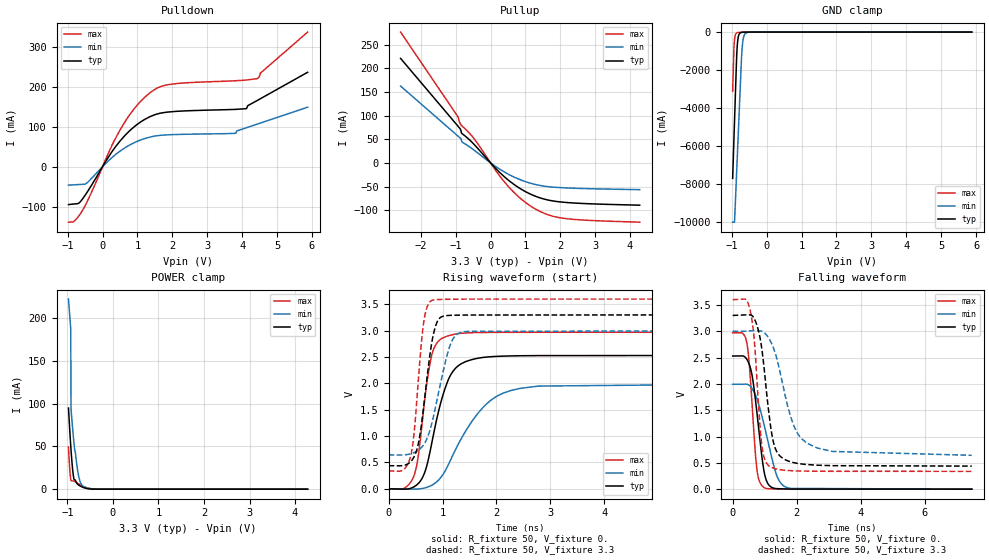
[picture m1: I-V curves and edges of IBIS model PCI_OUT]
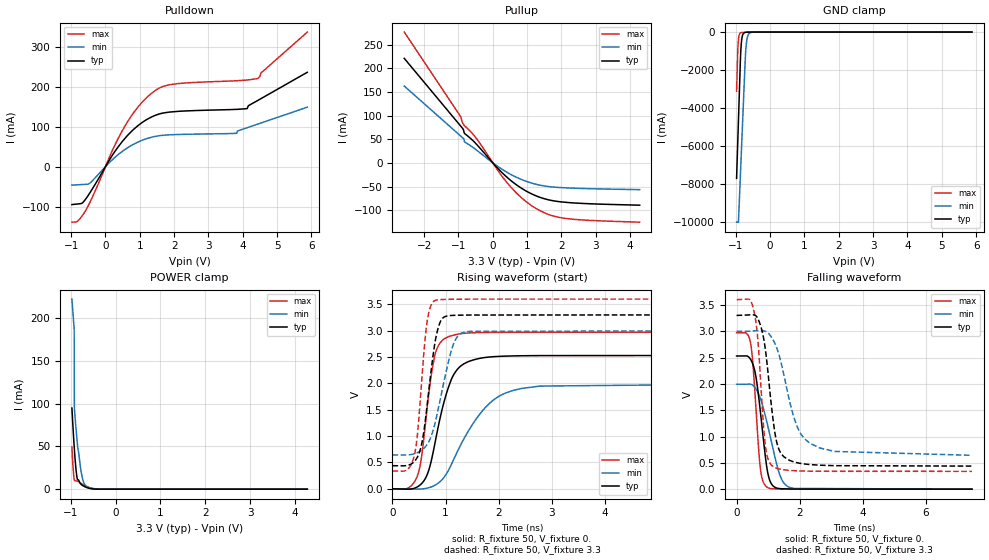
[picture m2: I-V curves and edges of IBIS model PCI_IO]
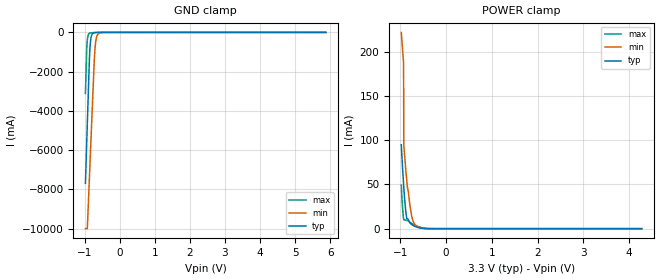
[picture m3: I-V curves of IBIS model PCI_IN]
|   IBIS Model for Tsi382 LQFP Package
[IBIS Ver]   3.2
[Disclaimer] This model is subject to change.
   Integrated Device Technology, Inc. ("IDT") hereby grants the
   user of this IBIS model a non-exclusive, nontransferable
   license to use this IBIS model under the following terms. The
   user is granted this license only to use the IBIS model and is
   not granted rights to sell, copy (except as needed to run the
   IBIS model), rent, lease or sub-license the IBIS model in
   whole or in part, or in modified form to anyone. The User may
   modify the IBIS model to suit its specific applications, but
   rights to derivative works and such modifications shall belong
   to IDT. This IBIS model is provided on an AS IS" basis and IDT
   makes absolutely no warranty with respect to the information
   contained herein. IDT DISCLAIMS AND CUSTOMER WAIVES ALL
   WARRANTIES, EXPRESS AND IMPLIED, INCLUDING WARRANTIES OF
   MERCHANTABILITY AND FITNESS FOR A PARTICULAR PURPOSE. THE
   ENTIRE RISK AS TO QUALITY AND PERFORMANCE IS WITH THE USER
   ACCORDINGLY, IN NO EVENT SHALL IDT BE LIABLE FOR ANY DIRECT OR
   INDIRECT DAMAGES, WHETHER IN CONTRACT OR TORT, INCLUDING ANY
   LOST PROFITS OR OTHER INCIDENTAL, CONSEQUENTIAL, EXEMPLARY, OR
   PUNITIVE DAMAGES ARISING OUT OF THE USE OR APPLICATION OF THE
   IBIS model. Further, IDT reserves the right to make changes
   without notice to any product herein to improve reliability,
   function, or design. IDT does not convey any license under
   patent rights or any other intellectual property rights,
   including those of third parties. IDT is not obligated to
   provide maintenance or support for the licensed IBIS model.
[Copyright]   Copyright 2009, Integrated Device Technology, Inc. all
   rights reserved.
[File Name]   tsi382_qfp.ibs
[File Rev]   1.3
[Notes]
   Revision History
   Rev 1.0
   - 07/17/2008 Inital Release. IBIS model generated from
   SPICE model extraction. IT
   Rev 1.1
   - 11/14/2008 - Updated 'model_name' definitions. IT
   Rev 1.2
   - 08/31/2009 - Updated with IDT formatting. IT
   Rev 1.3
   - 11/09/2009 Changed pin #136 from VDD_PCI to VIO_PCI.
[Component] Tsi382
[Manufacturer] Integrated Device Technology, Inc.
|   typ   min   max
[Package]
R_pkg   119m   116m   130m
L_pkg   7.62nH   7.61nH   8.82nH
C_pkg   0.52pF   0.46pF   0.59pF
[Pin]  signal_name   model_name   R_pin   L_pin   C_pin
6   GPIO[0]   NC   117.3m   7.7nh   0.52pf
11   GPIO[1]   NC   116.4m   7.6nh   0.52pf
9   GPIO[2]   NC   117.3m   7.7nh   0.52pf
10   GPIO[3]   NC   116.4m   7.7nh   0.53pf
97   JTAG_TCK   JTAG_IN   118.9m   7.9nh   0.54pf
98   JTAG_TDI   JTAG_IN   118.8m   7.5nh   0.54pf
86   JTAG_TDO   JTAG_OUT   132.9m   9.0nh   0.58pf
129   JTAG_TMS   JTAG_IN   128.3m   8.8nh   0.56pf
127   JTAG_TRSTn   JTAG_IN   125.0m   8.3nh   0.55pf
56   PCI_AD[0]   PCI_IO   119.0m   7.5nh   0.52pf
53   PCI_AD[1]   PCI_IO   122.1m   8.0nh   0.54pf
65   PCI_AD[10]   PCI_IO   119.3m   7.0nh   0.48pf
72   PCI_AD[11]   PCI_IO   118.1m   6.9nh   0.49pf
73   PCI_AD[12]   PCI_IO   118.6m   7.2nh   0.51pf
76   PCI_AD[13]   PCI_IO   121.1m   7.7nh   0.52pf
77   PCI_AD[14]   PCI_IO   121.2m   7.8nh   0.51pf
78   PCI_AD[15]   PCI_IO   121.0m   7.7nh   0.51pf
92   PCI_AD[16]   PCI_IO   126.0m   8.6nh   0.54pf
114   PCI_AD[17]   PCI_IO   117.8m   7.0nh   0.48pf
113   PCI_AD[18]   PCI_IO   117.6m   7.1nh   0.49pf
112   PCI_AD[19]   PCI_IO   118.8m   7.2nh   0.48pf
60   PCI_AD[2]   PCI_IO   118.4m   7.3nh   0.50pf
109   PCI_AD[20]   PCI_IO   117.0m   7.0nh   0.47pf
115   PCI_AD[21]   PCI_IO   116.8m   6.9nh   0.48pf
118   PCI_AD[22]   PCI_IO   117.4m   7.6nh   0.51pf
119   PCI_AD[23]   PCI_IO   116.6m   7.5nh   0.49pf
121   PCI_AD[24]   PCI_IO   116.3m   7.5nh   0.56pf
125   PCI_AD[25]   PCI_IO   121.1m   7.9nh   0.52pf
123   PCI_AD[26]   PCI_IO   119.7m   7.8nh   0.52pf
124   PCI_AD[27]   PCI_IO   118.9m   8.1nh   0.51pf
142   PCI_AD[28]   PCI_IO   120.1m   7.9nh   0.51pf
143   PCI_AD[29]   PCI_IO   119.6m   7.5nh   0.52pf
57   PCI_AD[3]   PCI_IO   119.3m   7.6nh   0.50pf
147   PCI_AD[30]   PCI_IO   116.8m   7.4nh   0.49pf
141   PCI_AD[31]   PCI_IO   119.7m   7.7nh   0.52pf
64   PCI_AD[4]   PCI_IO   119.3m   7.0nh   0.48pf
62   PCI_AD[5]   PCI_IO   118.0m   7.3nh   0.49pf
61   PCI_AD[6]   PCI_IO   117.5m   7.3nh   0.50pf
52   PCI_AD[7]   PCI_IO   122.3m   8.1nh   0.54pf
67   PCI_AD[8]   PCI_IO   121.1m   7.2nh   0.49pf
70   PCI_AD[9]   PCI_IO   119.2m   7.0nh   0.50pf
66   PCI_CBEn[0]   PCI_IO   121.0m   7.3nh   0.48pf
79   PCI_CBEn[1]   PCI_IO   122.2m   7.9nh   0.53pf
103   PCI_CBEn[2]   PCI_IO   114.7m   7.3nh   0.48pf
120   PCI_CBEn[3]   PCI_IO   115.7m   7.5nh   0.50pf
167   PCI_CLK   PCI_IN   122.5m   7.7nh   0.52pf
146   PCI_CLKO[0]   PCI_OUT   121.0m   7.3nh   0.50pf
51   PCI_CLKO[1]   PCI_OUT   124.8m   8.3nh   0.55pf
134   PCI_CLKO[2]   PCI_OUT   130.2m   8.9nh   0.57pf
137   PCI_CLKO[3]   PCI_OUT   123.0m   8.3nh   0.55pf
170   PCI_CLKO[4]   PCI_OUT   122.7m   7.8nh   0.54pf
96   PCI_DEVSELn   PCI_IO   120.0m   7.7nh   0.54pf
106   PCI_FRAMEn   PCI_IO   116.6m   7.2nh   0.46pf
152   PCI_GNTn[0]   PCI_IO   117.9m   6.8nh   0.76pf
155   PCI_GNTn[1]   PCI_OUT   118.8m   7.0nh   0.46pf
157   PCI_GNTn[2]   PCI_OUT   118.6m   6.9nh   0.60pf
163   PCI_GNTn[3]   PCI_OUT   118.4m   7.6nh   0.82pf
162   PCI_INTAn   PCI_IN   117.8m   7.5nh   0.54pf
161   PCI_INTBn   PCI_IN   118.1m   7.0nh   0.84pf
168   PCI_INTCn   PCI_IN   123.2m   7.9nh   0.75pf
164   PCI_INTDn   PCI_IN   119.1m   7.4nh   0.59pf
105   PCI_IRDYn   PCI_IO   115.7m   7.0nh   0.58pf
94   PCI_LOCKn   PCI_OUT   123.1m   8.2nh   0.48pf
169   PCI_M66EN   PCI_IN   124.3m   8.1nh   0.71pf
82   PCI_PAR   PCI_IO   128.8m   8.1nh   0.52pf
85   PCI_PERRn   PCI_IO   131.1m   8.7nh   0.84pf
149   PCI_PMEn   PCI_IN   119.0m   7.0nh   0.48pf
153   PCI_REQn[0]   PCI_IO   117.6m   6.9nh   0.62pf
138   PCI_REQn[1]   PCI_IN   121.8m   8.3nh   0.82pf
154   PCI_REQn[2]   PCI_IN   118.5m   6.9nh   0.52pf
148   PCI_REQn[3]   PCI_IN   119.0m   7.0nh   0.58pf
158   PCI_RSTn   PCI_OUT   118.6m   6.9nh   0.47pf
83   PCI_SERRn   PCI_IO   130.0m   8.6nh   0.48pf
102   PCI_STOPn   PCI_IO   114.1m   7.4nh   0.92pf
104   PCI_TRDYn   PCI_IO   115.4m   7.4nh   0.53pf
174   PCIE_PERSTn   NC   133.3m   8.8nh   0.70pf
22   PCIE_REFCLK_n   NC   111.3m   6.6nh   0.40pf
21   PCIE_REFCLK_p   NC   111.7m   6.6nh   0.39pf
24   PCIE_REXT   NC   111.3m   6.8nh   0.75pf
26   PCIE_RXD_n   NC   108.5m   6.6nh   0.45pf
27   PCIE_RXD_p   NC   107.0m   6.6nh   0.41pf
30   PCIE_TXD_n   NC   105.5m   7.0nh   0.41pf
29   PCIE_TXD_p   NC   105.7m   6.9nh   0.39pf
140   PWRUP_EN_ARB   GEN33_IN   119.7m   7.7nh   0.52pf
93   PWRUP_PLL_BYPASS   GEN33_IN   126.0m   8.6nh   0.54pf
48   SR_CLK   NC   132.9m   8.7nh   0.54pf
38   SR_CSn   NC   110.9m   7.5nh   0.51pf
37   SR_DIN   NC   111.8m   7.5nh   0.51pf
47   SR_DOUT   NC   132.9m   8.7nh   0.54pf
15   TEST_BCE   NC   117.0m   7.0nh   0.46pf
49   TEST_BIDR_CTL   NC   130.1m   8.6nh   0.55pf
35   TEST_ON   NC   107.2m   7.2nh   0.57pf
128   TEST_SPARE[0]   NC   126.7m   8.5nh   0.57pf
12   TEST_SPARE[1]   NC   116.8m   7.4nh   0.51pf
84   TEST_SPARE[2]   NC   130.0m   8.8nh   0.56pf
7   VDD   POWER
36   VDD   POWER
58   VDD   POWER
74   VDD   POWER
108   VDD   POWER
130   VDD   POWER
144   VDD   POWER
159   VDD   POWER
54   VDD_PCI   POWER
68   VDD_PCI   POWER
80   VDD_PCI   POWER
100   VDD_PCI   POWER
116   VDD_PCI   POWER
150   VDD_PCI   POWER
166   VDD_PCI   POWER
172   VDD_PCI   POWER
18   VDD_PCIE   POWER
33   VDD_PCIE   POWER
19   VDDA_PCIE   POWER
32   VDDA_PCIE   POWER
14   VDDA_PLL   POWER
71   VIO_PCI   POWER
111   VIO_PCI   POWER
136   VIO_PCI   POWER
173   VIO_PCI   POWER
1   VSS   GND
2   VSS   GND
3   VSS   GND
4   VSS   GND
5   VSS   GND
8   VSS   GND
13   VSS   GND
17   VSS   GND
20   VSS   GND
23   VSS   GND
25   VSS   GND
28   VSS   GND
31   VSS   GND
34   VSS   GND
39   VSS   GND
40   VSS   GND
41   VSS   GND
42   VSS   GND
43   VSS   GND
44   VSS   GND
45   VSS   GND
46   VSS   GND
50   VSS   GND
55   VSS   GND
59   VSS   GND
63   VSS   GND
69   VSS   GND
75   VSS   GND
81   VSS   GND
87   VSS   GND
88   VSS   GND
89   VSS   GND
90   VSS   GND
91   VSS   GND
95   VSS   GND
99   VSS   GND
101   VSS   GND
107   VSS   GND
110   VSS   GND
117   VSS   GND
122   VSS   GND
126   VSS   GND
131   VSS   GND
132   VSS   GND
133   VSS   GND
135   VSS   GND
139   VSS   GND
145   VSS   GND
151   VSS   GND
156   VSS   GND
160   VSS   GND
165   VSS   GND
171   VSS   GND
175   VSS   GND
176   VSS   GND
16   VSSA_PLL   GND
| Models and submodels in the file (6): PCI_OUT (Output), PCI_IO (I/O), PCI_IN (Input), JTAG_IN (Input), JTAG_OUT (Output), GEN33_IN (Input)
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[Model]   PCI_OUT
Model_type  Output
C_comp 4.536p 4.202p 4.874p
Polarity   Non-Inverting
Enable   Active-High
Vmeas =   1.32V
Cref =   10pF
Rref =   50
Vref=   0.0V
[Temperature Range]   27.0   125.0   -40.0
[Voltage Range] 3.3 3. 3.6
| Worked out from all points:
|   slope of the pulldown table from 0 to 0.495 V, typ, clamps not added: 7.81 ohm
|   slope of the pullup table from 0 to 0.495 V, typ, clamps not added: 13.9 ohm
|   GND clamp passes 1 mA (typ) near -0.58 V on its own axis
|   POWER clamp passes 1 mA (typ) near -0.59 V on its own axis
|   rising waveform, R_fixture 50, V_fixture 0.: 20-80 % time 365ps typ, 723ps min, 222ps max; typ from 0 V to 2.53 V
|   rising waveform, R_fixture 50, V_fixture 3.3: 20-80 % time 214ps typ, 317ps min, 159ps max; typ from 0.438 V to 3.3 V
|   falling waveform, R_fixture 50, V_fixture 0.: 20-80 % time 295ps typ, 484ps min, 203ps max; typ from 2.53 V to 0 V
|   falling waveform, R_fixture 50, V_fixture 3.3: 20-80 % time 338ps typ, 623ps min, 226ps max; typ from 3.3 V to 0.438 V
[Pulldown]
-976.9mV  -94.66mA   -46.06mA   -138.7mA
-817.5mV  -93.23mA   -45.29mA   -136.5mA
-595.7mV  -83.14mA   -44.21mA   -112.2mA
-429.3mV  -61.97mA   -39.17mA   -84.92mA
492.7mV   63.11mA    38.33mA    90.31mA
936.3mV   101.8mA    61.1mA     147.9mA
1.352V    124.6mA    73.73mA    184.1mA
1.851V    136.3mA    79.48mA    204.5mA
3.82V     143.1mA    83.35mA    214.6mA
4.125V    144.9mA    97.25mA    216.4mA
4.43V     165.1mA    106.2mA    220mA
5.879V    235.8mA    148.6mA    336.1mA
[Pullup]
-2.579V   220.8mA    162.3mA    276.3mA
-929mV    77.21mA    56.24mA    96.97mA
-887.4mV  73.58mA    53.57mA    85.73mA
-838.9mV  65.18mA    49.35mA    79.56mA
-818.1mV  61.78mA    43.99mA    77.84mA
-471.5mV  38.99mA    26.83mA    51.07mA
277.2mV   -21.28mA   -14.01mA   -29.14mA
623.8mV   -42.97mA   -28.22mA   -58.92mA
942.6mV   -58.4mA    -38.19mA   -80.33mA
1.442V    -74.52mA   -48.11mA   -103.5mA
1.969V    -82.31mA   -52.22mA   -115.7mA
4.277V    -89.5mA    -56.68mA   -125.4mA
[GND Clamp]
-976.9mV  -7.694A    -10A       -3.11A
-940.4mV  -5.645A    -10A       -848.5mA
-923.3mV  -4.682A    -10A       -400.9mA
-899.6mV  -3.359A    -8.991A    -148.3mA
-863.2mV  -1.353A    -7.407A    -43.18mA
-837.4mV  -553.5mA   -6.29A     -25.04mA
-794.5mV  -126.9mA   -4.431A    -15.74mA
-727.9mV  -18.49mA   -1.562A    -9.993mA
-708.6mV  -11.57mA   -935.5mA   -8.672mA
-670mV    -5.111mA   -330.6mA   -6.269mA
-603.5mV  -1.592mA   -60.06mA   -2.971mA
5.879V    0A         0A         0A
[Power Clamp]
-976.9mV  94.83mA    222.1mA    49.21mA
-949.3mV  68.95mA    202.6mA    23.59mA
-927.1mV  50.38mA    187.5mA    11.34mA
-921.6mV  46.09mA    93.87mA    10.01mA
-888.4mV  24.44mA    72.65mA    9.649mA
-855.2mV  11.42mA    53.18mA    9.29mA
-783.3mV  6.267mA    24.59mA    7.167mA
-750.1mV  4.693mA    14.57mA    6.03mA
-705.8mV  3.303mA    6.993mA    4.715mA
-656.1mV  2.103mA    3.495mA    3.408mA
-357.3mV  8.391uA    72.94uA    14.41uA
4.277V    0A         0A         0A
[Ramp]
dV/dt_r 1.518/365.23p 1.196/721.023p 1.782/221.8p
dV/dt_f 1.717/337.435p 1.415/622.991p 1.957/226.082p
[Rising Waveform]
R_fixture = 50
V_fixture = 0.
0s        0V         0V         0V
470ps     37.05mV    -6.726mV   246.6mV
550ps     99.96mV    -3.323mV   620.7mV
650ps     259.3mV    11.36mV    1.507V
800ps     863.9mV    67.25mV    2.539V
1.05ns    1.912V     341.7mV    2.883V
1.27ns    2.315V     802.2mV    2.942V
1.67ns    2.48V      1.449V     2.965V
2.28ns    2.522V     1.869V     2.969V
7.47ns    2.529V     1.993V     2.97V
[Rising Waveform]
R_fixture = 50
V_fixture = 3.3
V_fixture_min = 3.
V_fixture_max = 3.6
0s        438.2mV    642.1mV    338.6mV
410ps     515.4mV    664.5mV    626mV
470ps     601.9mV    685.9mV    1.029V
550ps     848.7mV    731.3mV    2.042V
650ps     1.557V     836.6mV    3.151V
800ps     2.767V     1.238V     3.573V
930ps     3.219V     1.841V     3.591V
1.13ns    3.29V      2.691V     3.596V
1.35ns    3.296V     2.969V     3.599V
7.47ns    3.3V       3V         3.6V
[Falling Waveform]
R_fixture = 50
V_fixture = 0.
0s        2.529V     1.993V     2.97V
440ps     2.469V     1.994V     2.787V
510ps     2.384V     1.976V     2.438V
600ps     2.182V     1.917V     1.677V
760ps     1.445V     1.712V     366.7mV
980ps     340.4mV    1.227V     32.06mV
1.12ns    87.95mV    862.5mV    8.858mV
1.38ns    10.32mV    256.9mV    3.596mV
1.74ns    3.211mV    22.96mV    1.388mV
7.47ns    1.068uV    15.07uV    0V
[Falling Waveform]
R_fixture = 50
V_fixture = 3.3
V_fixture_min = 3.
V_fixture_max = 3.6
0s        3.3V       3V         3.6V
420ps     3.311V     3.001V     3.601V
560ps     3.308V     3.009V     3.356V
680ps     3.232V     3.01V      2.799V
910ps     2.668V     3V         845.2mV
1.15ns    1.357V     2.845V     435.1mV
1.44ns    655.6mV    2.332V     374.1mV
1.88ns    507.9mV    1.256V     349.5mV
2.32ns    467.9mV    874.5mV    342.5mV
7.47ns    438.2mV    643.1mV    338.6mV
[Model]   PCI_IO
Model_type  I/O
C_comp 4.536p 4.202p 4.874p
Polarity   Non-Inverting
Enable   Active-High
Vinl =   0.80V
Vinh =   2.00V
Vmeas =   1.32V
Cref =   10pF
Rref =   50
Vref=   0.0V
[Temperature Range]   27.0   125.0   -40.0
[Voltage Range] 3.3 3. 3.6
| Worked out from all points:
|   slope of the pulldown table from 0 to 0.495 V, typ, clamps not added: 7.81 ohm
|   slope of the pullup table from 0 to 0.495 V, typ, clamps not added: 13.9 ohm
|   GND clamp passes 1 mA (typ) near -0.58 V on its own axis
|   POWER clamp passes 1 mA (typ) near -0.59 V on its own axis
|   rising waveform, R_fixture 50, V_fixture 0.: 20-80 % time 365ps typ, 723ps min, 222ps max; typ from 0 V to 2.53 V
|   rising waveform, R_fixture 50, V_fixture 3.3: 20-80 % time 214ps typ, 317ps min, 159ps max; typ from 0.438 V to 3.3 V
|   falling waveform, R_fixture 50, V_fixture 0.: 20-80 % time 295ps typ, 484ps min, 203ps max; typ from 2.53 V to 0 V
|   falling waveform, R_fixture 50, V_fixture 3.3: 20-80 % time 338ps typ, 623ps min, 226ps max; typ from 3.3 V to 0.438 V
[Pulldown]
-976.9mV  -94.66mA   -46.06mA   -138.7mA
-817.5mV  -93.23mA   -45.29mA   -136.5mA
-595.7mV  -83.14mA   -44.21mA   -112.2mA
-429.3mV  -61.97mA   -39.17mA   -84.92mA
492.7mV   63.11mA    38.33mA    90.31mA
936.3mV   101.8mA    61.1mA     147.9mA
1.352V    124.6mA    73.73mA    184.1mA
1.851V    136.3mA    79.48mA    204.5mA
3.82V     143.1mA    83.35mA    214.6mA
4.125V    144.9mA    97.25mA    216.4mA
4.43V     165.1mA    106.2mA    220mA
5.879V    235.8mA    148.6mA    336.1mA
[Pullup]
-2.579V   220.8mA    162.3mA    276.3mA
-929mV    77.21mA    56.24mA    96.97mA
-887.4mV  73.58mA    53.57mA    85.73mA
-838.9mV  65.18mA    49.35mA    79.56mA
-818.1mV  61.78mA    43.99mA    77.84mA
-471.5mV  38.99mA    26.83mA    51.07mA
277.2mV   -21.28mA   -14.01mA   -29.14mA
623.8mV   -42.97mA   -28.22mA   -58.92mA
942.6mV   -58.4mA    -38.19mA   -80.33mA
1.442V    -74.52mA   -48.11mA   -103.5mA
1.969V    -82.31mA   -52.22mA   -115.7mA
4.277V    -89.5mA    -56.68mA   -125.4mA
[GND Clamp]
-976.9mV  -7.694A    -10A       -3.11A
-940.4mV  -5.645A    -10A       -848.5mA
-923.3mV  -4.682A    -10A       -400.9mA
-899.6mV  -3.359A    -8.991A    -148.3mA
-863.2mV  -1.353A    -7.407A    -43.18mA
-837.4mV  -553.5mA   -6.29A     -25.04mA
-794.5mV  -126.9mA   -4.431A    -15.74mA
-727.9mV  -18.49mA   -1.562A    -9.993mA
-708.6mV  -11.57mA   -935.5mA   -8.672mA
-670mV    -5.111mA   -330.6mA   -6.269mA
-603.5mV  -1.592mA   -60.06mA   -2.971mA
5.879V    0A         0A         0A
[Power Clamp]
-976.9mV  94.83mA    222.1mA    49.21mA
-949.3mV  68.95mA    202.6mA    23.59mA
-927.1mV  50.38mA    187.5mA    11.34mA
-921.6mV  46.09mA    93.87mA    10.01mA
-888.4mV  24.44mA    72.65mA    9.649mA
-855.2mV  11.42mA    53.18mA    9.29mA
-783.3mV  6.267mA    24.59mA    7.167mA
-750.1mV  4.693mA    14.57mA    6.03mA
-705.8mV  3.303mA    6.993mA    4.715mA
-656.1mV  2.103mA    3.495mA    3.408mA
-357.3mV  8.391uA    72.94uA    14.41uA
4.277V    0A         0A         0A
[Ramp]
dV/dt_r 1.518/365.23p 1.196/721.023p 1.782/221.8p
dV/dt_f 1.717/337.435p 1.415/622.991p 1.957/226.082p
[Rising Waveform]
R_fixture = 50
V_fixture = 0.
0s        0V         0V         0V
470ps     37.05mV    -6.726mV   246.6mV
550ps     99.96mV    -3.323mV   620.7mV
650ps     259.3mV    11.36mV    1.507V
800ps     863.9mV    67.25mV    2.539V
1.05ns    1.912V     341.7mV    2.883V
1.27ns    2.315V     802.2mV    2.942V
1.67ns    2.48V      1.449V     2.965V
2.28ns    2.522V     1.869V     2.969V
7.47ns    2.529V     1.993V     2.97V
[Rising Waveform]
R_fixture = 50
V_fixture = 3.3
V_fixture_min = 3.
V_fixture_max = 3.6
0s        438.2mV    642.1mV    338.6mV
410ps     515.4mV    664.5mV    626mV
470ps     601.9mV    685.9mV    1.029V
550ps     848.7mV    731.3mV    2.042V
650ps     1.557V     836.6mV    3.151V
800ps     2.767V     1.238V     3.573V
930ps     3.219V     1.841V     3.591V
1.13ns    3.29V      2.691V     3.596V
1.35ns    3.296V     2.969V     3.599V
7.47ns    3.3V       3V         3.6V
[Falling Waveform]
R_fixture = 50
V_fixture = 0.
0s        2.529V     1.993V     2.97V
440ps     2.469V     1.994V     2.787V
510ps     2.384V     1.976V     2.438V
600ps     2.182V     1.917V     1.677V
760ps     1.445V     1.712V     366.7mV
980ps     340.4mV    1.227V     32.06mV
1.12ns    87.95mV    862.5mV    8.858mV
1.38ns    10.32mV    256.9mV    3.596mV
1.74ns    3.211mV    22.96mV    1.388mV
7.47ns    1.068uV    15.07uV    0V
[Falling Waveform]
R_fixture = 50
V_fixture = 3.3
V_fixture_min = 3.
V_fixture_max = 3.6
0s        3.3V       3V         3.6V
420ps     3.311V     3.001V     3.601V
560ps     3.308V     3.009V     3.356V
680ps     3.232V     3.01V      2.799V
910ps     2.668V     3V         845.2mV
1.15ns    1.357V     2.845V     435.1mV
1.44ns    655.6mV    2.332V     374.1mV
1.88ns    507.9mV    1.256V     349.5mV
2.32ns    467.9mV    874.5mV    342.5mV
7.47ns    438.2mV    643.1mV    338.6mV
|   MODEL PCI_IN
[Model]   PCI_IN
Model_type  Input
C_comp 4.536p 4.202p 4.874p
Polarity   Non-Inverting
Enable   Active-High
Vinl =   0.80V
Vinh =   2.00V
[Temperature Range]   27.0   125.0   -40.0
[POWER Clamp Reference]   3.30V   3.00V   3.60V
[GND Clamp Reference]   0.00V   0.00V   0.00V
[Voltage Range] 3.3 3. 3.6
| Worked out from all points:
|   GND clamp passes 1 mA (typ) near -0.58 V on its own axis
|   POWER clamp passes 1 mA (typ) near -0.59 V on its own axis
[GND Clamp]
-976.9mV  -7.694A    -10A       -3.11A
-940.4mV  -5.645A    -10A       -848.5mA
-923.3mV  -4.682A    -10A       -400.9mA
-899.6mV  -3.359A    -8.991A    -148.3mA
-863.2mV  -1.353A    -7.407A    -43.18mA
-837.4mV  -553.5mA   -6.29A     -25.04mA
-794.5mV  -126.9mA   -4.431A    -15.74mA
-727.9mV  -18.49mA   -1.562A    -9.993mA
-708.6mV  -11.57mA   -935.5mA   -8.672mA
-670mV    -5.111mA   -330.6mA   -6.269mA
-603.5mV  -1.592mA   -60.06mA   -2.971mA
5.879V    0A         0A         0A
[Power Clamp]
-976.9mV  94.83mA    222.1mA    49.21mA
-949.3mV  68.95mA    202.6mA    23.59mA
-927.1mV  50.38mA    187.5mA    11.34mA
-921.6mV  46.09mA    93.87mA    10.01mA
-888.4mV  24.44mA    72.65mA    9.649mA
-855.2mV  11.42mA    53.18mA    9.29mA
-783.3mV  6.267mA    24.59mA    7.167mA
-750.1mV  4.693mA    14.57mA    6.03mA
-705.8mV  3.303mA    6.993mA    4.715mA
-656.1mV  2.103mA    3.495mA    3.408mA
-357.3mV  8.391uA    72.94uA    14.41uA
4.277V    0A         0A         0A
